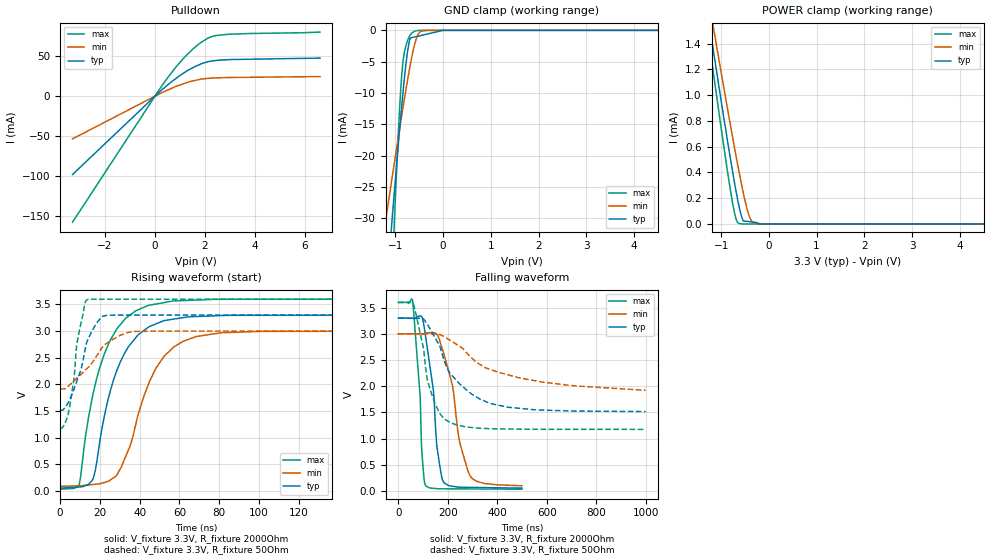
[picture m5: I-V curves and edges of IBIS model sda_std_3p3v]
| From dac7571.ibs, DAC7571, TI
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|   SDA_3p3V standard mode IO OPEN DRAIN MODEL
|   3.3v freq-400k,Rload=2Kohm, Cload = 15pF
[Model]   sda_std_3p3v
Model_type   I/O_open_drain
Polarity   Non-Inverting
Enable   Active-Low
Vinl = 0.99
Vinh = 2.31
Vmeas = 1.65
Vref = 3.3
Cref = 15pF
Rref = 2000
|   typ   min   max
|   (nom PVT)   (Fast PVT)   (Slow PVT)
|Average
C_comp   4.960e-12   4.955e-12   4.980e-12
|ON state : BUFFER OUTPUT TURNED LOW
|C_comp   5.983e-10   5.025e-10   5.601e-10
|OFF state : BUFFER IN HIGH IMPEDANCE STATE
|C_comp   4.960e-12   4.980e-12   4.955e-12
|Where nom PVT is NOM Process, 3.3V,25C
|   Fast PVT is Strong Process, 3.6V, -40C
|   Slow PVT is Weak Process, 3.0V, 105C
[Model spec]
|   typ   min   max
Vinl   0.99   0.9   1.08
Vinh   2.31   2.1   2.52
[Voltage Range]   3.3   3   3.6
[Temperature Range]   25   105   -40
|Junction temperature
[Pullup Reference]   3.3   3   3.6
[Pulldown Reference]   0   0   0
[Power Clamp Reference]   3.3   3   3.6
[GND Clamp Reference]   0   0   0
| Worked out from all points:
|   slope of the pulldown table from 0 to 0.495 V, typ, clamps not added: 36.2 ohm
|   GND clamp passes 1 mA (typ) near -0.56 V on its own axis
|   POWER clamp passes 1 mA (typ) near -1.02 V on its own axis
|   falling waveform, V_fixture 3.3V, R_fixture 2000Ohm: 20-80 % time 41ns typ, 67.3ns min, 24.4ns max; typ from 3.3 V to 0.056 V
|   rising waveform, V_fixture 3.3V, R_fixture 2000Ohm: 20-80 % time 14.4ns typ, 17.1ns min, 14.3ns max; typ from 0.055 V to 3.3 V
|   falling waveform, V_fixture 3.3V, R_fixture 50Ohm: 20-80 % time 143ns typ, 275ns min, 66.1ns max; typ from 3.3 V to 1.52 V
|   rising waveform, V_fixture 3.3V, R_fixture 50Ohm: 20-80 % time 8.68ns typ, 15.1ns min, 5.17ns max; typ from 1.52 V to 3.3 V
[Pulldown]
|   Voltage   I(typ)   I(min)   I(max)
-3.3V     -97.88mA   -53.33mA   -157.4mA
318mV     9.006mA    5.005mA    14.9mA
876mV     22.96mA    12.66mA    37.86mA
1.204V    29.99mA    16.21mA    49.42mA
1.52V     35.68mA    19.08mA    59.08mA
1.826V    40.06mA    21.19mA    66.83mA
2.266V    43.78mA    22.62mA    74.33mA
2.946V    45.58mA    23.31mA    77.37mA
6.6V      47.55mA    24.48mA    80.03mA
[GND Clamp]
|   Voltage   I(typ)   I(min)   I(max)
-3.3V     -246.7mA   -140.1mA   -463.1mA
-1.269V   -49.35mA   -33.72mA   -76.76mA
-1.208V   -43.43mA   -30.6mA    -65.2mA
-1.072V   -30.43mA   -23.65mA   -39.58mA
-1.047V   -28.13mA   -22.41mA   -35.08mA
-1.021V   -25.74mA   -21.13mA   -30.4mA
-916.8mV  -16.27mA   -15.97mA   -13.2mA
-844.8mV  -10.23mA   -12.5mA    -5.268mA
-719.4mV  -2.164mA   -6.811mA   -1.175mA
-618mV    -1.095mA   -2.867mA   -222.2uA
-330mV    -584.6uA   -3.168uA   -32.31nA
6.6V      0A         0A         0A
[POWER Clamp]
|   Voltage   I(typ)   I(min)   I(max)
-3.3V     6.651mA    6.278mA    7.033mA
-1.313V   1.712mA    1.855mA    1.577mA
-1.247V   1.552mA    1.712mA    1.401mA
-1.154V   1.327mA    1.51mA     1.152mA
-873.6mV  662.5uA    910uA      425.5uA
-762mV    411.2uA    678.4uA    166.8uA
-690mV    259.4uA    532.3uA    42.61uA
-621.6mV  131.7uA    399.4uA    2.885uA
-534.6mV  22.99uA    239.9uA    49.46nA
-411mV    17.67uA    60.06uA    38nA
-261mV    11.22uA    1.335uA    24.09nA
6.6V      0A         0A         0A
[Ramp]
R_load = 2000
|   typ   min   max
dV/dt_r   1.94677/1.43449e-08   1.74602/1.6822e-08   2.13769/1.41994e-08
dV/dt_f   1.94165/4.04541e-08   1.65863/6.17516e-08   2.13731/2.42467e-08
[Falling Waveform]
V_fixture = 3.3V
V_fixture_min = 3V
V_fixture_max = 3.6V
R_fixture = 2000Ohm
|   Time   V(typ)   V(min)   V(max)
0s        3.3V       3V         3.6V
58.07ns   3.3V       3V         3.632V
88.45ns   3.341V     3V         1.812V
95.65ns   3.323V     3V         731.8mV
110.9ns   2.94V      3.01V      105.5mV
142.8ns   1.899V     3.025V     53.39mV
157ns     826mV      2.982V     46.75mV
183.8ns   168.8mV    2.624V     44.19mV
287ns     71.71mV    321.7mV    41.91mV
500ns     56.49mV    102.2mV    37.22mV
[Rising Waveform]
V_fixture = 3.3V
V_fixture_min = 3V
V_fixture_max = 3.6V
R_fixture = 2000Ohm
|   Time   V(typ)   V(min)   V(max)
0s        55.39mV    89.97mV    37.18mV
9.565ns   78.19mV    100.2mV    120.4mV
16.3ns    216mV      124mV      1.778V
23.39ns   1.606V     175.3mV    2.676V
27.95ns   2.205V     278.1mV    3.005V
35.35ns   2.754V     868.3mV    3.306V
44.04ns   3.063V     1.968V     3.477V
57.25ns   3.225V     2.704V     3.565V
81.17ns   3.29V      2.969V     3.595V
300ns     3.3V       3V         3.6V
[Falling Waveform]
V_fixture = 3.3V
V_fixture_min = 3V
V_fixture_max = 3.6V
R_fixture = 50Ohm
|   Time   V(typ)   V(min)   V(max)
0s        3.3V       3V         3.6V
60.09ns   3.295V     3V         3.582V
102.5ns   3.282V     3V         2.715V
114.2ns   3.206V     3V         2.222V
125.5ns   3.12V      3V         1.997V
164.1ns   2.8V       2.989V     1.516V
206.7ns   2.267V     2.887V     1.316V
326.7ns   1.765V     2.427V     1.201V
443.5ns   1.6V       2.218V     1.185V
1us       1.518V     1.923V     1.178V
[Rising Waveform]
V_fixture = 3.3V
V_fixture_min = 3V
V_fixture_max = 3.6V
R_fixture = 50Ohm
|   Time   V(typ)   V(min)   V(max)
0s        1.517V     1.917V     1.178V
4.161ns   1.665V     1.971V     1.466V
6.945ns   1.913V     2.065V     2.108V
8.11ns    2.032V     2.107V     2.665V
8.719ns   2.095V     2.128V     2.821V
12.43ns   2.636V     2.26V      3.521V
14.23ns   2.862V     2.324V     3.596V
21.31ns   3.278V     2.702V     3.596V
36.74ns   3.3V       2.993V     3.596V
300ns     3.3V       3V         3.6V
